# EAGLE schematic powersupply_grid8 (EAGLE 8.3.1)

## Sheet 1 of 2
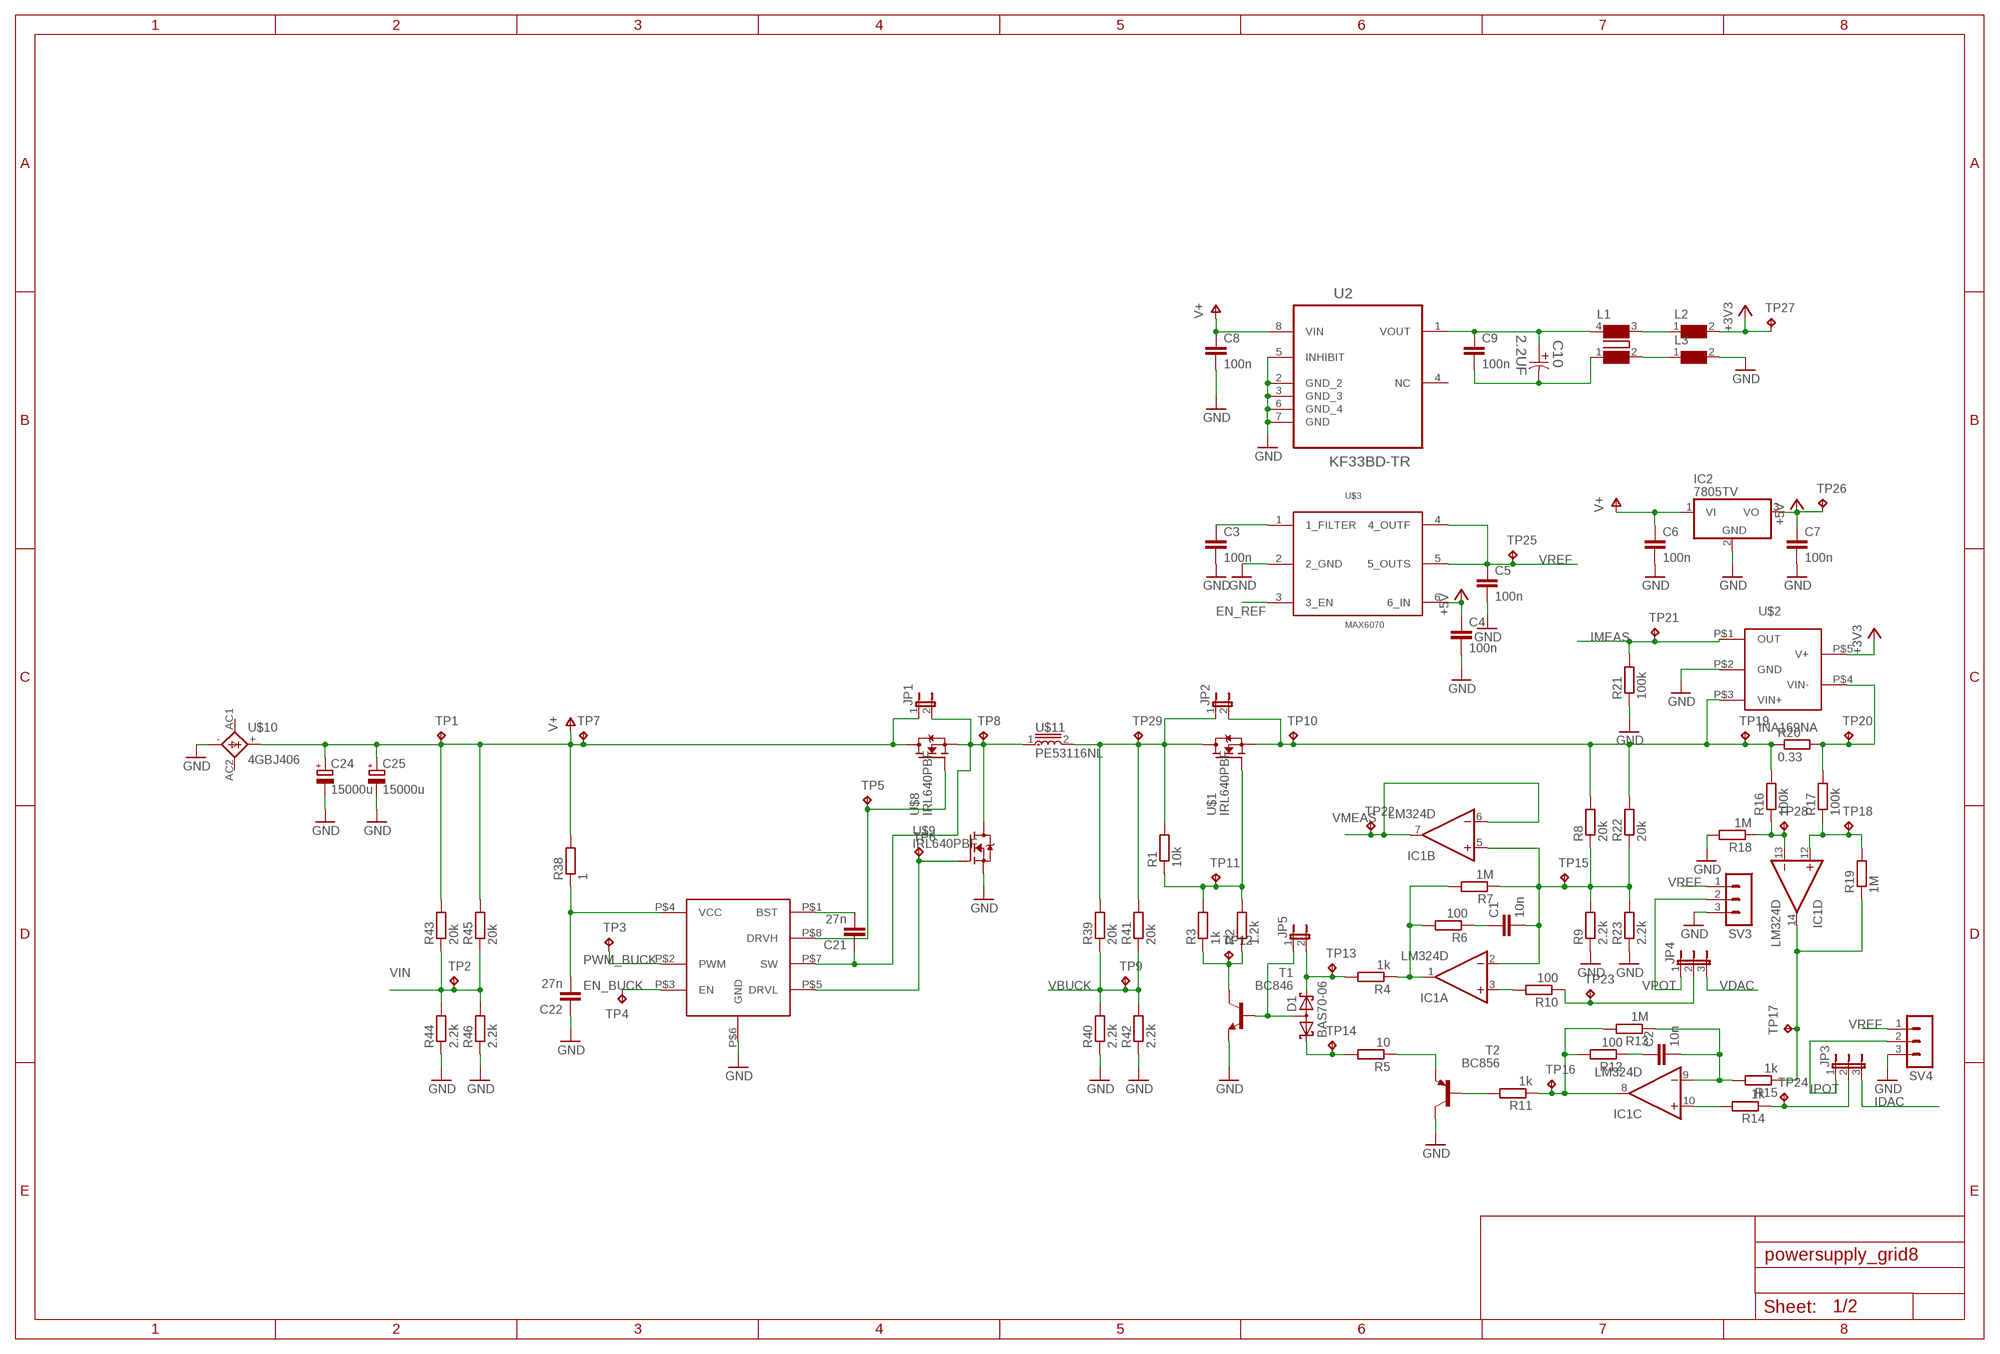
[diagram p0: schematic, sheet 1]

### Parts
C1  10n  C-EUC0805  [C0805]
C2  10n  C-EUC0805  [C0805]
C3  100n  C-EUC0402  [C0402]
C4  100n  C-EUC0402  [C0402]
C5  100n  C-EUC0402  [C0402]
C6  100n  C-EUC0402  [C0402]
C7  100n  C-EUC0402  [C0402]
C8  100n  C-EUC0603  [C0603]
C9  100n  C-EUC0603  [C0603]
C10  2.2UF  EEE-HB1H2R2R-CASE-B  [CAPAE430X610N]
C21  27n  C-EUC0805  [C0805]
C22  27n  C-EUC0805  [C0805]
C24  15000u  CPOL-EUE10-30  [EB30D]
C25  15000u  CPOL-EUE10-30  [EB30D]
D1  BAS70-06  [SOT23]
IC1  LM324D  [SO14]
IC2  7805TV  [TO220V]
JP1  JP1E  [JP1]
JP2  JP1E  [JP1]
JP3  JP2E  [JP2]
JP4  JP2E  [JP2]
JP5  JP1E  [JP1]
L1  WE-CNSW-744232222_1206  [WE-CNSW_1206]
L2  WE-CBF-742792042_0805  [0805]
L3  WE-CBF-742792042_0805  [0805]
R1  10k  R-EU_R0805  [R0805]
R2  1.2k  R-EU_R0805  [R0805]
R3  1k  R-EU_R0805  [R0805]
R4  1k  R-EU_R0805  [R0805]
R5  10  R-EU_R0805  [R0805]
R6  100  R-EU_R0805  [R0805]
R7  1M  R-EU_R0805  [R0805]
R8  20k  R-EU_R0805  [R0805]
R9  2.2k  R-EU_R0805  [R0805]
R10  100  R-EU_R0805  [R0805]
R11  1k  R-EU_R0805  [R0805]
R12  100  R-EU_R0805  [R0805]
R13  1M  R-EU_R0805  [R0805]
R14  1k  R-EU_R0805  [R0805]
R15  1k  R-EU_R0805  [R0805]
R16  100k  R-EU_R0805  [R0805]
R17  100k  R-EU_R0805  [R0805]
R18  1M  R-EU_R0805  [R0805]
R19  1M  R-EU_R0805  [R0805]
R20  0.33  R-EU_R2010  [R2010]
R21  100k  R-EU_R0805  [R0805]
R22  20k  R-EU_R0805  [R0805]
R23  2.2k  R-EU_R0805  [R0805]
R38  1  R-EU_R0805  [R0805]
R39  20k  R-EU_R0805  [R0805]
R40  2.2k  R-EU_R0805  [R0805]
R41  20k  R-EU_R0805  [R0805]
R42  2.2k  R-EU_R0805  [R0805]
R43  20k  R-EU_R0805  [R0805]
R44  2.2k  R-EU_R0805  [R0805]
R45  20k  R-EU_R0805  [R0805]
R46  2.2k  R-EU_R0805  [R0805]
SV3  MA03-1  [MA03-1]
SV4  MA03-1  [MA03-1]
T1  BC846  [SOT23]
T2  BC856  BC856A-PNP-SOT23-BEC  [SOT23-BEC]
TP1  TPB2,54  [B2,54]
TP2  TPB2,54  [B2,54]
TP3  TPB2,54  [B2,54]
TP4  TPB2,54  [B2,54]
TP5  TPB2,54  [B2,54]
TP6  TPB2,54  [B2,54]
TP7  TPB2,54  [B2,54]
TP8  TPB2,54  [B2,54]
TP9  TPB2,54  [B2,54]
TP10  TPB2,54  [B2,54]
TP11  TPB2,54  [B2,54]
TP12  TPB2,54  [B2,54]
TP13  TPB2,54  [B2,54]
TP14  TPB2,54  [B2,54]
TP15  TPB2,54  [B2,54]
TP16  TPB2,54  [B2,54]
TP17  TPB2,54  [B2,54]
TP18  TPB2,54  [B2,54]
TP19  TPB2,54  [B2,54]
TP20  TPB2,54  [B2,54]
TP21  TPB2,54  [B2,54]
TP22  TPB2,54  [B2,54]
TP23  TPB2,54  [B2,54]
TP24  TPB2,54  [B2,54]
TP25  TPB2,54  [B2,54]
TP26  TPB2,54  [B2,54]
TP27  TPB2,54  [B2,54]
TP28  TPB2,54  [B2,54]
TP29  TPB2,54  [B2,54]
U2  KF33BD-TR  [SOIC127P600X175-8N]
U$1  IRL640PBF  [TO-220AB]
U$2  INA169NA  [SOT23]
U$3  MAX6070  [SOT23-6]
U$7  NCP5901B  [SOIC-8]
U$8  IRL640PBF  [TO-220AB]
U$9  IRL640PBF  [TO-220AB]
U$10  4GBJ406  [FB100]
U$11  PE53116NL  [SFT1030]

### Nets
+3V3: L2.2 TP27.TP U$2.P$5(V+) ; also sheet 2
+5V: C4.1 C7.1 IC2.3(VO) TP26.TP U$3.6(6_IN) ; also sheet 2
EN_BUCK: TP4.TP U$7.P$3(EN)
EN_REF: U$3.3(3_EN)
GND: C3.2 C4.2 C5.2 C6.2 C7.2 C8.2 C22.1 C24.- C25.- IC2.2(GND) L3.2 R9.1 R18.2 R21.1 R23.1 R40.1 R42.1 R44.1 R46.1 SV3.3 SV4.3 T1.2(E) T2.C U2.2(GND_2) U2.3(GND_3) U2.5(INHIBIT) U2.6(GND_4) U2.7(GND) U$2.P$2(GND) U$3.2(2_GND) U$7.P$6(GND) U$9.P$3(S) U$10.- ; also sheet 2
IDAC: JP3.3 ; also sheet 2
IMEAS: R21.2 TP21.TP U$2.P$1(OUT) ; also sheet 2
IPOT: JP3.1 SV4.2
N$1: C9.1 C10.1 L1.4 U2.1(VOUT)
N$2: R1.1 R2.2 R3.2 TP11.TP U$1.P$1(G)
N$3: R2.1 R3.1 T1.3(C) TP12.TP
N$4: D1.3(AA) JP5.1 T1.1(B)
N$5: D1.2(K2) JP5.2 R4.2 TP13.TP
N$6: D1.1(K1) R5.2 TP14.TP
N$7: IC1.1(A:OUT) R4.1 R6.2 R7.2
N$8: C3.1 U$3.1(1_FILTER)
N$9: C1.1 R6.1
N$10: C1.2 IC1.2(A:-IN) IC1.5(B:+IN) R7.1 R8.1 R9.2 R22.1 R23.2 TP15.TP
N$11: JP2.2 R8.2 R16.2 R20.1 R22.2 TP10.TP TP19.TP U$1.P$3(S) U$2.P$3(VIN+)
N$12: R5.1 T2.E
N$13: IC1.3(A:+IN) R10.2
N$14: R11.2 T2.B
N$15: IC1.14(D:OUT) R15.1 R19.1 TP17.TP
N$16: IC1.8(C:OUT) R11.1 R12.2 R13.2 TP16.TP
N$17: C2.2 IC1.9(C:-IN) R13.1 R15.2
N$18: C2.1 R12.1
N$19: IC1.10(C:+IN) R14.2
N$20: IC1.13(D:-IN) R16.1 R18.1 TP28.TP
N$21: IC1.12(D:+IN) R17.1 R19.2 TP18.TP
N$22: R17.2 R20.2 TP20.TP U$2.P$4(VIN-)
N$23: L1.2 L3.1
N$24: L1.3 L2.1
N$25: C9.2 C10.2 L1.1
N$34: TP5.TP U$7.P$8(DRVH) U$8.P$1(G)
N$35: TP6.TP U$7.P$5(DRVL) U$9.P$1(G)
N$42: C21.2 U$7.P$1(BST)
N$43: JP2.1 R1.2 R39.2 R41.2 TP29.TP U$1.P$2(D) U$11.2
N$44: C22.2 R38.1 U$7.P$4(VCC)
N$47: JP3.2 R14.1 TP24.TP
N$48: JP4.2 R10.1 TP23.TP
N$49: C21.1 JP1.2 TP8.TP U$7.P$7(SW) U$8.P$3(S) U$9.P$2(D) U$11.1
PWM_BUCK: TP3.TP U$7.P$2(PWM) ; also sheet 2
V+: C6.1 C8.1 C24.+ C25.+ IC2.1(VI) JP1.1 R38.2 R43.2 R45.2 TP1.TP TP7.TP U2.8(VIN) U$8.P$2(D) U$10.+
VBUCK: R39.1 R40.2 R41.1 R42.2 TP9.TP ; also sheet 2
VDAC: JP4.3 ; also sheet 2
VIN: R43.1 R44.2 R45.1 R46.2 TP2.TP ; also sheet 2
VMEAS: IC1.6(B:-IN) IC1.7(B:OUT) TP22.TP ; also sheet 2
VPOT: JP4.1 SV3.2
VREF: C5.1 SV3.1 SV4.1 TP25.TP U$3.4(4_OUTF) U$3.5(5_OUTS) ; also sheet 2
Unconnected: U2.4(NC) U$10.AC1 U$10.AC2

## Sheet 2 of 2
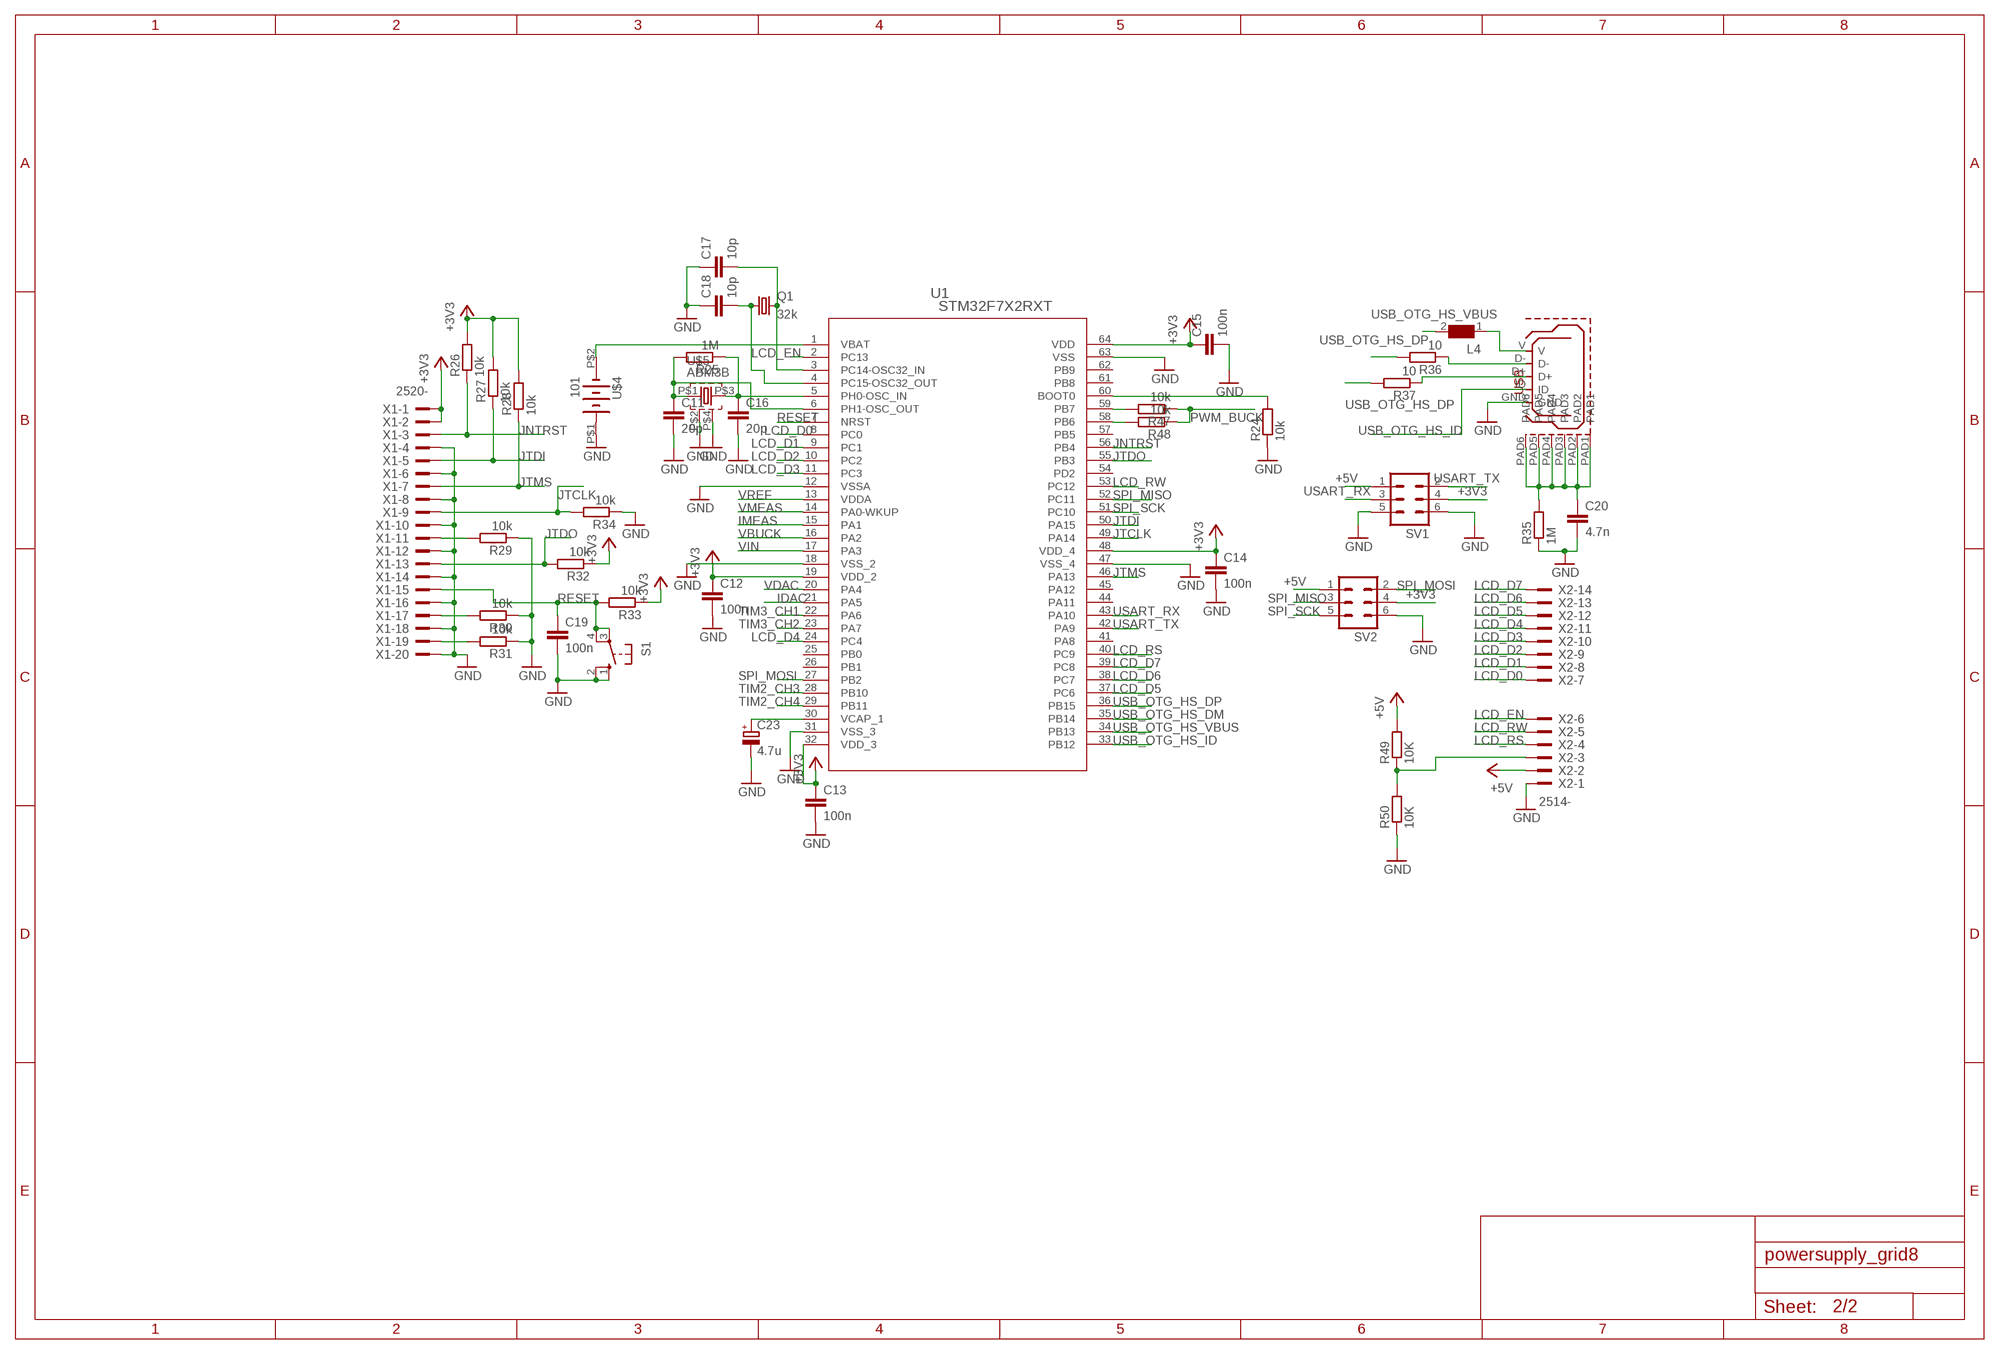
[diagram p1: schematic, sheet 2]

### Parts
C11  20p  C-EUC0402  [C0402]
C12  100n  C-EUC0402  [C0402]
C13  100n  C-EUC0603  [C0603]
C14  100n  C-EUC0402  [C0402]
C15  100n  C-EUC0402  [C0402]
C16  20p  C-EUC0402  [C0402]
C17  10p  C-EUC0402  [C0402]
C18  10p  C-EUC0402  [C0402]
C19  100n  C-EUC0402  [C0402]
C20  4.7n  C-EUC0805  [C0805]
C23  4.7u  CPOL-EUE2.5-7  [E2,5-7]
L4  WE-CBF-742792641_0603  [0603]
Q1  32k  CRYSTALTC26V  [TC26V]
R24  10k  R-EU_R0805  [R0805]
R25  1M  R-EU_R0402  [R0402]
R26  10k  R-EU_R0805  [R0805]
R27  10k  R-EU_R0805  [R0805]
R28  10k  R-EU_R0805  [R0805]
R29  10k  R-EU_R0805  [R0805]
R30  10k  R-EU_R0805  [R0805]
R31  10k  R-EU_R0805  [R0805]
R32  10k  R-EU_R0805  [R0805]
R33  10k  R-EU_R0805  [R0805]
R34  10k  R-EU_R0805  [R0805]
R35  1M  R-EU_R0805  [R0805]
R36  10  R-EU_R0805  [R0805]
R37  10  R-EU_R0805  [R0805]
R47  10k  R-EU_R0805  [R0805]
R48  10k  R-EU_R0805  [R0805]
R49  10K  R-EU_R0805  [R0805]
R50  10K  R-EU_R0805  [R0805]
S1  10-XX  [B3F-10XX]
SV1  ML6  [ML6]
SV2  ML6  [ML6]
U1  STM32F7X2RXT  [LQFP64-10X10MM]
U$4  101  [KEYSTONE101]
U$5  ABM3B  [ABM3B]
U$6  USB_MICROB  [USB_MICROB_PACKAGE]
X1  2520-  [PAK100/2500-20]
X2  2514-  [PAK100/2500-14]

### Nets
+3V3: C12.1 C13.1 C14.1 C15.1 R26.2 R27.2 R28.2 R32.1 R33.1 SV1.4 SV2.4 U1.19(VDD_2) U1.32(VDD_3) U1.48(VDD_4) U1.64(VDD) X1.1 X1.2 ; also sheet 1
+5V: R49.2 SV1.1 SV2.1 X2.2 ; also sheet 1
GND: C11.2 C12.2 C13.2 C14.2 C15.2 C16.2 C17.1 C18.1 C19.2 C20.2 C23.- R24.1 R29.1 R30.1 R31.1 R34.1 R35.1 R50.1 S1.1(S) S1.2(S1) SV1.5 SV1.6 SV2.6 U1.12(VSSA) U1.18(VSS_2) U1.31(VSS_3) U1.47(VSS_4) U1.63(VSS) U$4.P$1(+) U$5.P$2 U$5.P$4 U$6.GND X1.4 X1.6 X1.8 X1.10 X1.12 X1.14 X1.16 X1.18 X1.20 X2.1 ; also sheet 1
IDAC: U1.21(PA5) ; also sheet 1
IMEAS: U1.15(PA1) ; also sheet 1
JNTRST: R26.1 U1.56(PB4) X1.3
JTCLK: R34.2 U1.49(PA14) X1.9
JTDI: R27.1 U1.50(PA15) X1.5
JTDO: R32.2 U1.55(PB3) X1.13
JTMS: R28.1 U1.46(PA13) X1.7
LCD_D0: U1.8(PC0) X2.7
LCD_D1: U1.9(PC1) X2.8
LCD_D2: U1.10(PC2) X2.9
LCD_D3: U1.11(PC3) X2.10
LCD_D4: U1.24(PC4) X2.11
LCD_D5: U1.37(PC6) X2.12
LCD_D6: U1.38(PC7) X2.13
LCD_D7: U1.39(PC8) X2.14
LCD_EN: U1.2(PC13) X2.6
LCD_RS: U1.40(PC9) X2.4
LCD_RW: U1.53(PC12) X2.5
N$26: R24.2 U1.60(BOOT0)
N$27: U1.1(VBAT) U$4.P$2(-)
N$28: C16.1 R25.1 U1.5(PH0-OSC_IN) U$5.P$3
N$29: C11.1 R25.2 U1.6(PH1-OSC_OUT) U$5.P$1
N$30: C18.2 Q1.1 U1.4(PC15-OSC32_OUT)
N$31: C17.2 Q1.2 U1.3(PC14-OSC32_IN)
N$32: R29.2 X1.11
N$33: C20.1 R35.2 U$6.PAD1 U$6.PAD2 U$6.PAD3 U$6.PAD4 U$6.PAD5 U$6.PAD6
N$36: R30.2 X1.17
N$37: R31.2 X1.19
N$38: L4.1 U$6.V
N$39: R47.2 U1.59(PB7)
N$40: R36.1 U$6.D-
N$41: R37.1 U$6.D+
N$45: R48.2 U1.58(PB6)
N$46: C23.+ U1.30(VCAP_1)
N$50: R49.1 R50.2 X2.3
PWM_BUCK: R47.1 R48.1 ; also sheet 1
RESET: C19.1 R33.2 S1.3(P) S1.4(P1) U1.7(NRST) X1.15
SPI_MISO: SV2.3 U1.52(PC11)
SPI_MOSI: SV2.2 U1.27(PB2)
SPI_SCK: SV2.5 U1.51(PC10)
TIM2_CH3: U1.28(PB10)
TIM2_CH4: U1.29(PB11)
TIM3_CH1: U1.22(PA6)
TIM3_CH2: U1.23(PA7)
USART_RX: SV1.3 U1.43(PA10)
USART_TX: SV1.2 U1.42(PA9)
USB_OTG_HS_DM: U1.35(PB14)
USB_OTG_HS_DP: R36.2 R37.2 U1.36(PB15)
USB_OTG_HS_ID: U1.33(PB12) U$6.ID
USB_OTG_HS_VBUS: L4.2 U1.34(PB13)
VBUCK: U1.16(PA2) ; also sheet 1
VDAC: U1.20(PA4) ; also sheet 1
VIN: U1.17(PA3) ; also sheet 1
VMEAS: U1.14(PA0-WKUP) ; also sheet 1
VREF: U1.13(VDDA) ; also sheet 1
Unconnected: U1.25(PB0) U1.26(PB1) U1.41(PA8) U1.44(PA11) U1.45(PA12) U1.54(PD2) U1.57(PB5) U1.61(PB8) U1.62(PB9)

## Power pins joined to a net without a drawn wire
V+: IC1.4(P:V+)
V-: IC1.11(P:V-)

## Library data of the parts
C1-C9 C11-C22 = rcl:C-EU: CAPACITOR, European symbol; SPICEPREFIX: C
C10 = Panasonic-EEEFT_EEEH:EEE-: Aluminum Electrolytic Capacitors,Surface Mount Type; MPN: EEE-HB1H2R2R; OC_FARNELL: 9696865; OC_NEWARK: 96K9421; PACKAGE: CASE-B; SUPPLIER: PANASONIC; TOLERANCE: ±20 %; VOLTAGERATING: 50V
C23-C25 = rcl:CPOL-EU: POLARIZED CAPACITOR, European symbol
D1 = diode:BAS70-06: Silicon Schottky Diodes General-purpose diode for high-speed switching
IC1 = linear:LM324: OP AMP
IC2 = linear:78*: Positive VOLTAGE REGULATOR Source: http://cache.national.com/ds/LM/LM78L05.pdf http://www.fairchildsemi.com/ds/LM/LM7805.pdf
JP1 JP2 JP5 = jumper:JP1E: JUMPER
JP3 JP4 = jumper:JP2E: JUMPER
L1 = WE-CNSW:WE-CNSW: SMD Common Mode Noise Suppressor WE-CNSW - High common mode suppression at high frequency - Small influence for high speed signals through winding symmetry -- USB 2.0 -- Firewire / IEEE 1394 -- Power supply systems -- High Speed Data Lines -- Common mode data line filter; MPN: 744232222; OC_FARNELL: 1636481; OC_NEWARK: 08P2550; PACKAGE: 1206; SUPPLIER: WURTH ELEKTRONIK
L2 L3 = WE-CBF:WE-CBF: SMD EMI Suppression Ferrite Beads WE-CBF; MPN: 742792042; OC_FARNELL: 1635716; OC_NEWARK: 08P2373; PACKAGE: IND-0805; SUPPLIER: Wuerth Elektronik
L4 = WE-CBF:WE-CBF: SMD EMI Suppression Ferrite Beads WE-CBF; MPN: 742792641; OC_FARNELL: 1635705; OC_NEWARK: 08P2436; PACKAGE: IND-0603; SUPPLIER: Wuerth Elektronik
Q1 = crystal:CRYSTAL: CRYSTAL; OC_FARNELL: unknown; OC_NEWARK: unknown
R1-R50 = rcl:R-EU_: RESISTOR, European symbol; SPICEPREFIX: R
S1 = switch-omron:10-XX: OMRON SWITCH; MPN: B3F-1000; OC_FARNELL: 176432; OC_NEWARK: 36M3542
SV1 SV2 = con-harting-ml:ML6: HARTING; OC_FARNELL: unknown; OC_NEWARK: unknown
SV3 SV4 = con-lstb:MA03-1: PIN HEADER; OC_FARNELL: unknown; OC_NEWARK: unknown
T1 = transistor:BC846: NPN TRANSISTOR
T2 = transistor:*-PNP-: PNP Transistror
TP1-TP29 = testpad:TP: Test pad
U1 = STM32F732RE:STM32F7X2RXT; MANUFACTURER_PART_NUMBER: stm32f7x2rxt; VENDOR: STMicroelectronics
U2 = KF33BD-TR:KF33BD-TR: LDO, 0.4VDO, 0.5A, 3.3V, 2%, 8SOIC; MPN: KF33BD-TR; OC_FARNELL: 2253497; OC_NEWARK: 25M9948; PACKAGE: SOIC-8; SUPPLIER: STMicroelectronics
U$1 U$8 U$9 = TO-220AB:IRL640PBF
U$2 = INA169NA:INA169NA
U$3 = max6070:MAX6070
U$4 = my_battery:101
U$5 = crystal_my:ABM3B
U$6 = usb_hinrose:USB_MICROB: This is the hirose ZX62-B-5PA(11) MICRO-USB B Type female connection.
U$7 = NCP5901B:NCP5901B: The NCP5901B is a high performance dual MOSFET gate driver optimized to drive the gates of both high−side and low−side power MOSFETs in a synchronous buck converter.
U$10 = 4GBJ406F:4GBJ406
U$11 = PE53116NL:PE53116NL
X1 = con-3m:2520-: 3M (TM) Pak 100 4-Wall Header Source: 3M; OC_FARNELL: unknown; OC_NEWARK: unknown
X2 = con-3m:2514-: 3M (TM) Pak 100 4-Wall Header Source: 3M; OC_FARNELL: unknown; OC_NEWARK: unknown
